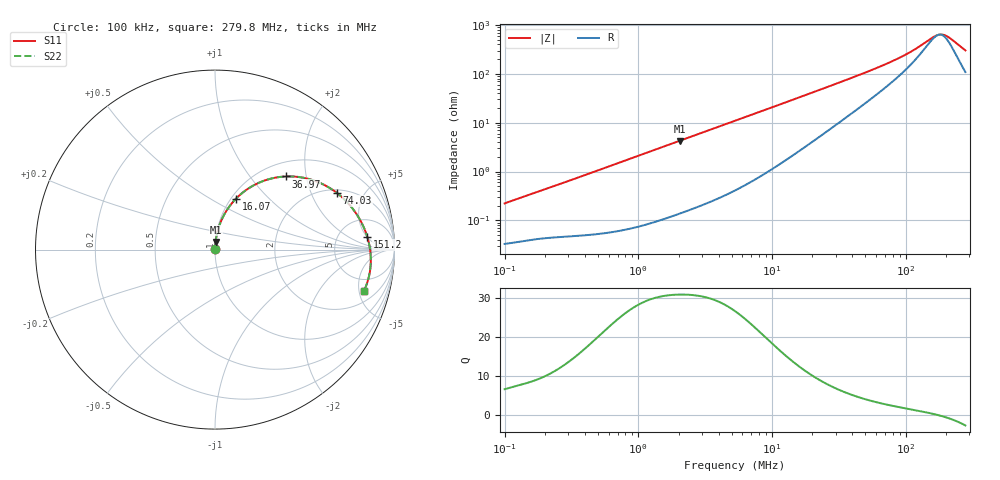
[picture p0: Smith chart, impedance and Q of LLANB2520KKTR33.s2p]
! LLANB2520KKTR33  S-PARAMETER MODEL  ( General Type )
! Model Generated by TAIYO YUDEN Corporation (http://www.ty-top.com)
! Version 2.0
! TAIYO YUDEN Control No. 20210629
! Copyright(c) 2016 TAIYO YUDEN CO.,LTD. All Rights Reserved.
! Product Description (link to TY-COMPAS)
! https://ds.yuden.co.jp/TYCOMPAS/or/detail?pn=LLANB2520KKTR33M&u=M
! Products Name : Inductors
! Characteristics :
!  Inductance : 0.33 uH , SRF(min) : -Hz , DC Resistance(max) : 0.038 Ohm
!  Rated Current : Saturation :4700 mA , Temp Rise : 3500 mA (40 degC)
!  Case Size : 2.5 x 2.0 / 0.098 x 0.079 [mm/inch] , Thickness : 1 / 0.039 [mm/inch]
!  (Conditions: Temperature = 25 degC , DC Bias Current/Voltage = 0A / 0V)
! External Node Assignments :
!  1  o---GGG---o  2
! GND o---------o GND
! Frequency Range : 0.1MHz  -  279.750408MHz  [ 402 STEP ]
# MHz S RI R 50
! Freq[MHz].  S11 Real  S11 Imag  S21 Real  S21 Imag  S12 Real  S12 Imag  S22 Real  S22 Imag
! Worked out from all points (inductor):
!   401 points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, 100 kHz to 279.8 MHz, reference 50 ohm
!   read as one part in series: L = 348 nH near 104 kHz
!   highest Q = 31 at 2.041 MHz (marker M1), where L = 331 nH
!   self-resonance near 177.7 MHz
!   S11 on the Smith chart (normalised r, x): 100 kHz: 1.00, +0.00; 16.07 MHz: 1.05, +0.66; 36.97 MHz: 1.27, +1.53; 74.03 MHz: 2.17, +3.12; 151.2 MHz: 10, +5; 279.8 MHz: 3.18, -5.65
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0.1  0.000333 0.0022  0.9997 -0.0022  0.9997 -0.0022  0.000333 0.0022
0.377863  0.000551 0.00798  0.9994 -0.00798  0.9994 -0.00798  0.000551 0.00798
1.427803  0.00187 0.0298  0.9981 -0.0298  0.9981 -0.0298  0.00187 0.0298
2.04067  0.00316 0.0423  0.9968 -0.0423  0.9968 -0.0423  0.00316 0.0423
5.289144  0.0157 0.1069  0.9843 -0.1069  0.9843 -0.1069  0.0157 0.1069
9.979919  0.0501 0.1928  0.9499 -0.1928  0.9499 -0.1928  0.0501 0.1928
16.06694  0.1173 0.2841  0.8827 -0.2841  0.8827 -0.2841  0.1173 0.2841
19.9857  0.1686 0.3286  0.8314 -0.3286  0.8314 -0.3286  0.1686 0.3286
28.00317  0.2787 0.3858  0.7213 -0.3858  0.7213 -0.3858  0.2787 0.3858
36.96955  0.3933 0.4075  0.6067 -0.4075  0.6067 -0.4075  0.3933 0.4075
51.80026  0.5414 0.388  0.4586 -0.388  0.4586 -0.388  0.5414 0.388
74.03492  0.6798 0.3154  0.3202 -0.3154  0.3202 -0.3154  0.6798 0.3154
75.51853  0.6865 0.3101  0.3135 -0.3101  0.3135 -0.3101  0.6865 0.3101
90.28298  0.7415 0.2584  0.2585 -0.2584  0.2585 -0.2584  0.7415 0.2584
107.934  0.7873 0.1998  0.2127 -0.1998  0.2127 -0.1998  0.7873 0.1998
126.5009  0.8204 0.1423  0.1796 -0.1423  0.1796 -0.1423  0.8204 0.1423
151.2328  0.8485 0.0711  0.1515 -0.0711  0.1515 -0.0711  0.8485 0.0711
173.7659  0.8626 0.0102  0.1374 -0.0102  0.1374 -0.0102  0.8626 0.0102
191.8886  0.8675 -0.0363  0.1325 0.0363  0.1325 0.0363  0.8675 -0.0363
211.9014  0.8672 -0.0851  0.1328 0.0851  0.1328 0.0851  0.8672 -0.0851
268.8666  0.8396 -0.2083  0.1604 0.2083  0.1604 0.2083  0.8396 -0.2083
279.7504  0.8308 -0.2289  0.1692 0.2289  0.1692 0.2289  0.8308 -0.2289
